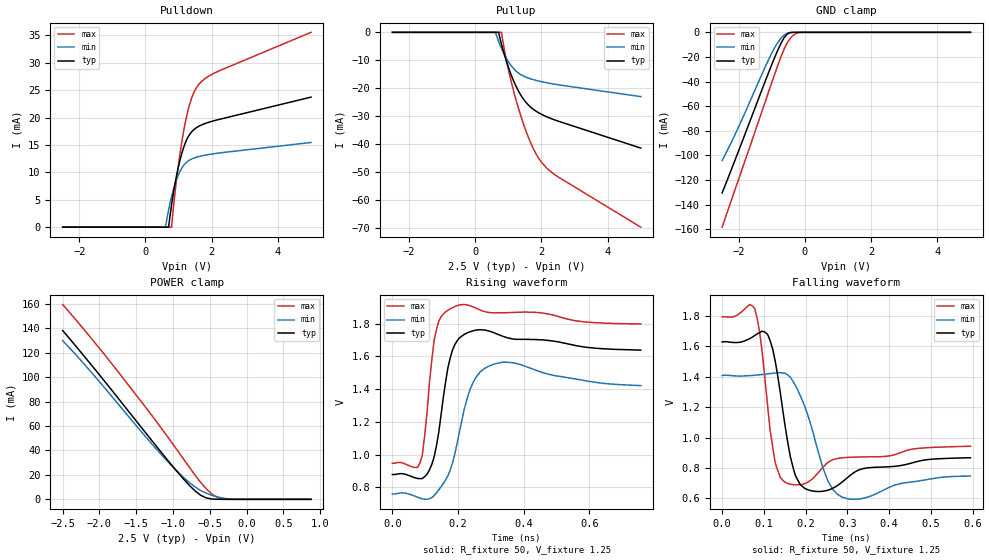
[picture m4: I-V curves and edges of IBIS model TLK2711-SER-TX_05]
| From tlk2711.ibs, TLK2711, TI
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|   Model TLK2711-SER-TX_05
[Model]   TLK2711-SER-TX_05
Model_type   3-state
Polarity   Non-Inverting
Enable   Active-Low
| Timing test load is based on data sheet information for rise and fall time
Vmeas = 1.25V
Cref  = 5pF
Rref  = 50Mohms
Vref  = 1.25V
| C_comp is estimated by modeling group by simulation
C_comp   0.9360pF   0.8158pF   0.9617pF
[Temperature Range]   27   85   -40
[Voltage Range]   2.5V   2.3V   2.7V
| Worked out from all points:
|   GND clamp passes 1 mA (typ) near -0.50 V on its own axis
|   POWER clamp passes 1 mA (typ) near -0.54 V on its own axis
|   rising waveform, R_fixture 50, V_fixture 1.25: 20-80 % time 33.8ps typ, 47.2ps min, 24.7ps max; typ from 0.878 V to 1.64 V
|   falling waveform, R_fixture 50, V_fixture 1.25: 20-80 % time 25.4ps typ, 45.8ps min, 19.5ps max; typ from 1.63 V to 0.867 V
[Pulldown]
| voltage   I(typ)   I(min)   I(max)
-2.5V     0A         0A         0A
600mV     5.79pA     2.02uA     0A
700mV     56.98uA    3.184mA    800fA
790mV     4.132mA    5.612mA    36.42uA
860mV     6.821mA    7.191mA    4.534mA
950mV     9.763mA    8.855mA    9.256mA
1.15V     14.49mA    11.26mA    17.44mA
1.325V    16.86mA    12.23mA    22.25mA
1.55V     18.21mA    12.79mA    25.58mA
1.775V    18.87mA    13.11mA    27.01mA
2.15V     19.56mA    13.48mA    28.33mA
5V        23.74mA    15.46mA    35.57mA
[Pullup]
| voltage   I(typ)   I(min)   I(max)
-2.5V     10.56nA    8.692nA    40.03nA
610mV     -23.82nA   -983.9nA   -32.1nA
710mV     -26.89uA   -3.333mA   -36.43nA
790mV     -4.097mA   -5.618mA   -2.251uA
890mV     -8.321mA   -8.126mA   -6.737mA
1.025V    -13.26mA   -10.87mA   -14.44mA
1.3V      -20.84mA   -14.49mA   -26.89mA
1.625V    -26.2mA    -16.43mA   -38.1mA
1.925V    -28.82mA   -17.44mA   -45.16mA
2.15V     -30.14mA   -18.01mA   -48.4mA
2.45V     -31.53mA   -18.64mA   -51.27mA
5V        -41.39mA   -22.98mA   -69.66mA
[GND_clamp]
| voltage   I(typ)   I(min)   I(max)
-2.5V     -130.6mA   -104.2mA   -158.4mA
-2.05V    -99.66mA   -79.61mA   -123.2mA
-1.225V   -41.59mA   -29.64mA   -58.49mA
-925mV    -21.19mA   -13.02mA   -34.91mA
-775mV    -11.89mA   -6.69mA    -23.59mA
-625mV    -4.281mA   -2.194mA   -13.44mA
-550mV    -1.797mA   -853.7uA   -9.328mA
-475mV    -515.9uA   -225.4uA   -6.047mA
-325mV    -16.34uA   -6.464uA   -1.843mA
-175mV    -335.2nA   -108.9nA   -179.3uA
-25mV     -17.29nA   -11.4nA    -5.392uA
5V        85.07nA    86.67nA    83.48nA
[POWER_clamp]
| voltage   I(typ)   I(min)   I(max)
-2.5V     138.1mA    129.8mA    159.4mA
-2.2V     116.5mA    110.1mA    138.2mA
-1.75V    83.01mA    78.25mA    104.6mA
-1.3V     48.95mA    46.12mA    69.52mA
-1V       26.62mA    26.3mA     44.98mA
-850mV    16.09mA    17.49mA    32.3mA
-700mV    6.829mA    10.06mA    19.69mA
-625mV    3.337mA    7.198mA    13.82mA
-475mV    282.6uA    3.358mA    4.459mA
-400mV    52.34uA    2.028mA    1.614mA
-250mV    1.171uA    360.3uA    76.11uA
875mV     0A         0A         0A
[Ramp]
| variable   typ   min   max
dV/dt_r 0.44898V/0.0324943ns  0.39072V/0.0465602ns  0.50364V/0.0239811ns
dV/dt_f 0.44856V/0.0249391ns  0.3891V/0.0451943ns  0.50334V/0.0186793ns
R_load = 50
[Rising Waveform]
R_fixture = 50
V_fixture = 1.25
V_fixture_min = 1.00
V_fixture_max = 1.40
| time   V(typ)   V(min)   V(max)
0s        877.7mV    758.8mV    946.6mV
84ps      852.5mV    733.9mV    949.9mV
98ps      864.2mV    726.9mV    1.11V
127ps     983.9mV    748.9mV    1.695V
148ps     1.238V     802.7mV    1.841V
176ps     1.589V     904.6mV    1.89V
197ps     1.694V     1.066V     1.91V
239ps     1.752V     1.409V     1.908V
295ps     1.754V     1.541V     1.868V
757ps     1.638V     1.421V     1.798V
[Falling Waveform]
R_fixture = 50
V_fixture = 1.25
V_fixture_min = 1.00
V_fixture_max = 1.40
| time   V(typ)   V(min)   V(max)
0s        1.628V     1.407V     1.792V
78ps      1.67V      1.409V     1.848V
90ps      1.69V      1.412V     1.69V
115ps     1.637V     1.42V      1.047V
127ps     1.505V     1.424V     836.1mV
151ps     1.073V     1.422V     705.8mV
187ps     690.9mV    1.277V     690mV
253ps     654mV      716.3mV    835.7mV
283ps     697.8mV    615.5mV    865.2mV
595ps     867.3mV    747mV      942.6mV
